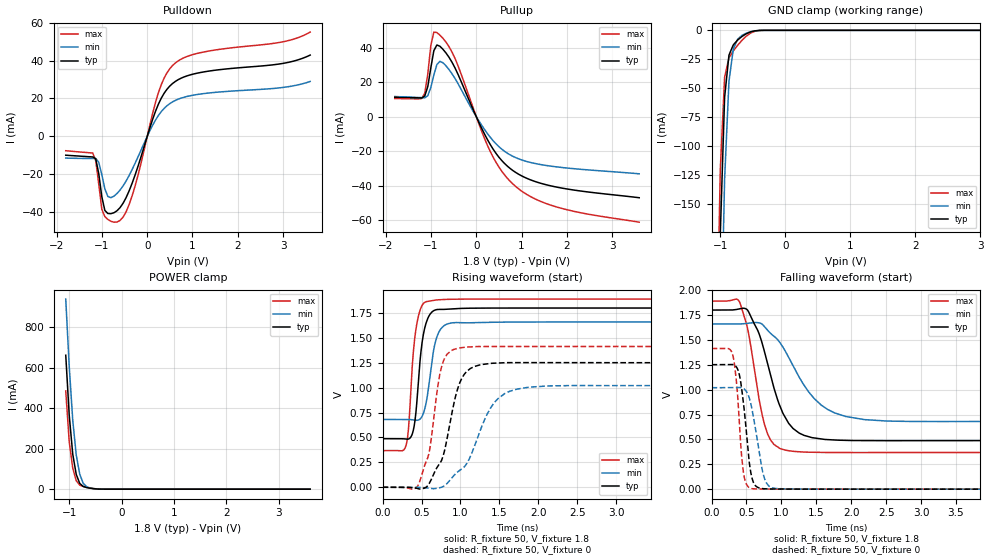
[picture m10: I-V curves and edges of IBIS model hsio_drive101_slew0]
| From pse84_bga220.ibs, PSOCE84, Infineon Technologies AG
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[Model] hsio_drive101_slew0
Model_type I/O
Enable   Active-High
Vinl  =  0.54
Vinh  =  1.26
Vmeas =  0.9
Cref  =  15pF
| Capacitance   typ   min   max
C_comp   1.183861e-12   1.145095e-12   1.230403e-12
| Variables   typ   min   max
[GND Clamp Reference]   0   0   0
[POWER Clamp Reference]   1.8   1.66   1.89
[Pulldown Reference]   0   0   0
[Pullup Reference]   1.8   1.66   1.89
[Temperature Range]   25   125   -40
[Voltage Range]   1.8   1.66   1.89
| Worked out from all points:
|   slope of the pulldown table from 0 to 0.27 V, typ, clamps not added: 14.9 ohm
|   slope of the pullup table from 0 to 0.27 V, typ, clamps not added: 18.8 ohm
|   GND clamp passes 1 mA (typ) near -0.51 V on its own axis
|   POWER clamp passes 1 mA (typ) near -0.47 V on its own axis
|   falling waveform, R_fixture 50, V_fixture 1.8: 20-80 % time 339ps typ, 533ps min, 226ps max; typ from 1.8 V to 0.488 V
|   falling waveform, R_fixture 50, V_fixture 0: 20-80 % time 111ps typ, 147ps min, 88.5ps max; typ from 1.25 V to 0 V
|   rising waveform, R_fixture 50, V_fixture 1.8: 20-80 % time 96.5ps typ, 114ps min, 87.3ps max; typ from 0.488 V to 1.8 V
|   rising waveform, R_fixture 50, V_fixture 0: 20-80 % time 225ps typ, 355ps min, 161ps max; typ from 0 V to 1.25 V
[GND Clamp]
| Voltage   I(typ)   I(min)   I(max)
-1.137V   -688mA     -831.1mA   -596.4mA
-1.07V    -398.5mA   -545.5mA   -312.5mA
-1.003V   -176.8mA   -300mA     -120.9mA
-936.6mV  -57.93mA   -128.6mA   -40.51mA
-869.7mV  -21.44mA   -44.12mA   -23.78mA
-802.8mV  -12.54mA   -16.03mA   -17.79mA
-735.9mV  -8.37mA    -7.69mA    -12.93mA
-669mV    -5.28mA    -4.356mA   -8.606mA
-535.2mV  -1.316mA   -1.208mA   -2.332mA
-401.4mV  -73.56uA   -132.2uA   -119.3uA
3.6V      0A         0A         0A
[POWER Clamp]
| Voltage   I(typ)   I(min)   I(max)
-1.07V    662.2mA    940mA      485.7mA
-1.003V   363.7mA    605.6mA    233mA
-936.6mV  172.7mA    341mA      103.9mA
-869.7mV  72.74mA    168.6mA    41.65mA
-802.8mV  28.31mA    73.56mA    19.99mA
-735.9mV  13.11mA    28.55mA    13.36mA
-669mV    7.76mA     11.5mA     8.963mA
-535.2mV  2.357mA    2.863mA    2.668mA
-334.5mV  34.33uA    127.4uA    15.59uA
3.6V      0A         0A         0A
[Pulldown]
| Voltage   I(typ)   I(min)   I(max)
-1.8V     -9.926mA   -11.45mA   -7.576mA
-1.204V   -10.85mA   -11.66mA   -8.775mA
-1.137V   -11.86mA   -11.66mA   -12.84mA
-1.003V   -31.78mA   -20.17mA   -38.45mA
-936.6mV  -39.04mA   -27.66mA   -42.31mA
-869.7mV  -40.68mA   -31.72mA   -43.81mA
-669mV    -39.25mA   -30.17mA   -45.18mA
-401.4mV  -28.82mA   -20.69mA   -36.06mA
248.3mV   17.05mA    11.05mA    23.1mA
558.6mV   27.85mA    18.19mA    37.33mA
1.117V    33.39mA    22.13mA    43.82mA
3.6V      42.87mA    28.96mA    54.99mA
[Pullup]
| Voltage   I(typ)   I(min)   I(max)
-1.8V     11.14mA    11.63mA    10.46mA
-1.204V   10.82mA    10.99mA    10.49mA
-1.137V   11.94mA    10.9mA     13.58mA
-1.07V    17.38mA    12.15mA    24.62mA
-1.003V   28.28mA    16.86mA    41.25mA
-936.6mV  38.22mA    24.15mA    48.98mA
-869.7mV  41.5mA     30.16mA    48.7mA
-468.3mV  28.17mA    22.07mA    33.67mA
310.3mV   -16.22mA   -11.99mA   -20.24mA
806.9mV   -31.21mA   -22.98mA   -38.99mA
1.738V    -40.65mA   -29.01mA   -52.08mA
3.6V      -47.02mA   -33.16mA   -61.2mA
[Ramp]
dV/dt_r   0.750667/0.225076n  0.611814/0.355291n  0.848063/0.16061n
dV/dt_f   0.787305/0.338634n  0.587327/0.532921n  0.913048/0.226006n
R_load = 50
[Falling Waveform]
R_fixture = 50
V_fixture = 1.8
V_fixture_min = 1.66
V_fixture_max = 1.89
| Time   V(typ)   V(min)   V(max)
0s        1.8V       1.66V      1.89V
376.7ps   1.808V     1.66V      1.904V
516.8ps   1.798V     1.666V     1.611V
691.9ps   1.54V      1.67V      860.3mV
802.2ps   1.259V     1.597V     554.9mV
1.023ns   761.4mV    1.427V     398.7mV
1.344ns   536.9mV    1.025V     372.3mV
1.763ns   493.7mV    766.3mV    368.1mV
2.811ns   487.4mV    680.7mV    368.3mV
50ns      487.8mV    681.1mV    368.3mV
[Falling Waveform]
R_fixture = 50
V_fixture = 0
V_fixture_min = 0
V_fixture_max = 0
| Time   V(typ)   V(min)   V(max)
0s        1.251V     1.02V      1.413V
286ps     1.253V     1.02V      1.383V
380.7ps   1.193V     1.022V     865.7mV
425.3ps   1.04V      1.02V      377.9mV
466.5ps   804.8mV    1.006V     127mV
549.7ps   219.2mV    893.2mV    11.21mV
624.7ps   38.13mV    622.5mV    2.564mV
780.7ps   3.137mV    69.94mV    1.041mV
1.102ns   684.5uV    2.555mV    307.1uV
50ns      12.84nV    968nV      4.63nV
[Rising Waveform]
R_fixture = 50
V_fixture = 1.8
V_fixture_min = 1.66
V_fixture_max = 1.89
| Time   V(typ)   V(min)   V(max)
0s        487.8mV    681.1mV    368.3mV
294.7ps   483.9mV    681.1mV    404.7mV
333.2ps   484.4mV    681.2mV    592.3mV
372.4ps   517.5mV    678.7mV    1.104V
443ps     881.7mV    672.7mV    1.654V
492ps     1.355V     693.7mV    1.801V
547.7ps   1.619V     805.4mV    1.86V
677.7ps   1.781V     1.457V     1.88V
811.5ps   1.788V     1.633V     1.887V
50ns      1.8V       1.66V      1.89V
[Rising Waveform]
R_fixture = 50
V_fixture = 0
V_fixture_min = 0
V_fixture_max = 0
| Time   V(typ)   V(min)   V(max)
0s        12.85nV    911.9nV    4.632nV
431.3ps   -8.785mV   -35.86uV   -5.681mV
579.6ps   15.5mV     -7.086mV   295.5mV
723.7ps   226.8mV    -6.651mV   1.087V
796.1ps   369mV      16.54mV    1.296V
990.7ps   1.049V     169.8mV    1.399V
1.199ns   1.217V     452.5mV    1.413V
1.484ns   1.248V     892.2mV    1.414V
2.141ns   1.251V     1.018V     1.413V
50ns      1.251V     1.02V      1.413V
